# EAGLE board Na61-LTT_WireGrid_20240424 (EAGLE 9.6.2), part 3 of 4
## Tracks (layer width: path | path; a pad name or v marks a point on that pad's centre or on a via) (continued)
S$3176 (continued)
  Bottom 0.152: 35.8,85 36.2,85
S$3177
  Bottom 0.152: 36.2,85 37.2,86
S$3178
  Bottom 0.152: 33.8,85 34.6,85
S$3179
  Bottom 0.152: 34.6,85 35.6,86
S$3180
  Bottom 0.152: 40.8,89 41.2,89.4
S$3181
  Bottom 0.152: 41.2,89.4 41.2,90
S$3182
  Bottom 0.152: 38.8,89 39.6,89.8
S$3183
  Bottom 0.152: 39.6,89.8 39.6,90
S$3184
  Bottom 0.152: 36.8,89 37,89
S$3185
  Bottom 0.152: 37,89 38,90
S$3186
  Bottom 0.152: 34.8,89 35.4,89
S$3187
  Bottom 0.152: 35.4,89 36.4,90
S$3188
  Bottom 0.152: 32.8,87 33.8,86
S$3189
  Bottom 0.152: 33.8,86 34.8,86
S$3190
  Bottom 0.152: 34.6,91 34,91
S$3191
  Bottom 0.152: 34,91 33,90
S$3192
  Bottom 0.152: 33,90 32.4,90
S$3193
  Bottom 0.152: 32.6,91 31.6,90
S$3194
  Bottom 0.152: 31.6,90 30.8,90
S$3195
  Bottom 0.152: 30.6,91 29.6,90
S$3196
  Bottom 0.152: 29.6,90 29.2,90
S$3197
  Bottom 0.152: 28.6,91 27.6,90
S$3198
  Bottom 0.152: 26.6,91 26,90.4
S$3199
  Bottom 0.152: 26,90.4 26,90
S$3200
  Bottom 0.152: 35.6,95 34.6,94
S$3201
  Bottom 0.152: 34.6,94 33.2,94
S$3202
  Bottom 0.152: 33.6,95 33.2,95
S$3203
  Bottom 0.152: 33.2,95 32.2,94
S$3204
  Bottom 0.152: 32.2,94 31.6,94
S$3205
  Bottom 0.152: 31.6,95 31,95
S$3206
  Bottom 0.152: 31,95 30,94
S$3207
  Bottom 0.152: 29.6,95 29.4,95
S$3208
  Bottom 0.152: 29.4,95 28.4,94
S$3209
  Bottom 0.152: 27.6,95 26.8,94.2
S$3210
  Bottom 0.152: 26.8,94.2 26.8,94
S$3211
  Bottom 0.152: 34,90 35.2,90
S$3212
  Bottom 0.152: 35.2,90 36.2,91
S$3213
  Bottom 0.152: 36.2,91 36.6,91
S$3214  (2 unrouted)
  Top 0.813: 65,94.5 65,85.5
  Top 1.8: 66,91.5 64,91.5 | 66,94.5 65,94.5 64,94.5 | 66,88.5 64,88.5 | 66,85.5 65,85.5 64,85.5
S$3215
  Top 1.778: -104.08,86.83 -104.08,88.35
S$3216
  Top 1.778: -104.08,91.65 -104.08,93.17
S$3217
  Top 1.778: -99,86.83 -99,88.35
S$3218
  Top 1.778: -99,91.65 -99,93.17
S$3219
  Top 1.778: -93.92,86.83 -93.92,88.35
S$3220
  Top 1.778: -93.92,91.65 -93.92,93.17
S$3221
  Top 1.778: 93.92,86.83 93.92,88.35
S$3222
  Top 1.778: 93.92,91.65 93.92,93.17
S$3223
  Top 1.778: 99,86.83 99,88.35
S$3224
  Top 1.778: 99,91.65 99,93.17
S$3225
  Top 1.778: 104.08,86.83 104.08,88.35
S$3226
  Top 1.778: 104.08,91.65 104.08,93.17
S$3235
  Bottom 0.8: 9.4,102.9 9.4,101.1
S$3236
  Bottom 0.8: 11.4,102.9 11.4,101.1
S$3237
  Bottom 0.8: 8.4,105.1 8.4,106.9
S$3238
  Bottom 0.8: 10.4,105.1 10.4,106.9
S$3239
  Bottom 0.8: 5.4,102.9 5.4,101.1
S$3240
  Bottom 0.8: 7.4,102.9 7.4,101.1
S$3241
  Bottom 0.8: 6.4,105.1 6.4,106.9
S$3242
  Bottom 0.8: 4.4,105.1 4.4,106.9
S$3243
  Bottom 0.8: 3.4,102.9 3.4,101.1
S$3244
  Bottom 0.8: 1.4,102.9 1.4,101.1
S$3245
  Bottom 0.8: 2.4,105.1 2.4,106.9
S$3246
  Bottom 0.8: 0.4,105.1 0.4,106.9
S$3247
  Bottom 0.8: -0.6,102.9 -0.6,101.1
S$3248
  Bottom 0.8: -2.6,102.9 -2.6,101.1
S$3249
  Bottom 0.8: -1.6,105.1 -1.6,106.9
S$3250
  Bottom 0.8: 17.4,102.9 17.4,101.1
S$3251
  Bottom 0.8: 19.4,102.9 19.4,101.1
S$3252
  Bottom 0.8: 16.4,105.1 16.4,106.9
S$3253
  Bottom 0.8: 18.4,105.1 18.4,106.9
S$3254
  Bottom 0.8: 13.4,102.9 13.4,101.1
S$3255
  Bottom 0.8: 15.4,102.9 15.4,101.1
S$3256
  Bottom 0.8: 12.4,105.1 12.4,106.9
S$3257
  Bottom 0.8: 14.4,105.1 14.4,106.9
S$3258
  Bottom 0.8: -7.4,110.9 -7.4,109.1
S$3259
  Bottom 0.8: -5.4,110.9 -5.4,109.1
S$3260
  Bottom 0.8: -8.4,113.1 -8.4,114.9
S$3261
  Bottom 0.8: -6.4,113.1 -6.4,114.9
S$3262
  Bottom 0.8: -11.4,110.9 -11.4,109.1
S$3263
  Bottom 0.8: -9.4,110.9 -9.4,109.1
S$3264
  Bottom 0.8: -10.4,113.1 -10.4,114.9
S$3265
  Bottom 0.8: -12.4,113.1 -12.4,114.9
S$3266
  Bottom 0.8: -13.4,110.9 -13.4,109.1
S$3267
  Bottom 0.8: -15.4,110.9 -15.4,109.1
S$3268
  Bottom 0.8: -14.4,113.1 -14.4,114.9
S$3269
  Bottom 0.8: -16.4,113.1 -16.4,114.9
S$3270
  Bottom 0.8: -17.4,110.9 -17.4,109.1
S$3271
  Bottom 0.8: -19.4,110.9 -19.4,109.1
S$3272
  Bottom 0.8: -18.4,113.1 -18.4,114.9
S$3273
  Bottom 0.8: 0.6,110.9 0.6,109.1
S$3274
  Bottom 0.8: 2.6,110.9 2.6,109.1
S$3275
  Bottom 0.8: -0.4,113.1 -0.4,114.9
S$3276
  Bottom 0.8: 1.6,113.1 1.6,114.9
S$3277
  Bottom 0.8: -3.4,110.9 -3.4,109.1
S$3278
  Bottom 0.8: -1.4,110.9 -1.4,109.1
S$3279
  Bottom 0.8: -4.4,113.1 -4.4,114.9
S$3280
  Bottom 0.8: -2.4,113.1 -2.4,114.9
S$3281
  Bottom 0.8: -24.6,102.9 -24.6,101.1
S$3282
  Bottom 0.8: -22.6,102.9 -22.6,101.1
S$3283
  Bottom 0.8: -25.6,105.1 -25.6,106.9
S$3284
  Bottom 0.8: -23.6,105.1 -23.6,106.9
S$3285
  Bottom 0.8: -28.6,102.9 -28.6,101.1
S$3286
  Bottom 0.8: -26.6,102.9 -26.6,101.1
S$3287
  Bottom 0.8: -27.6,105.1 -27.6,106.9
S$3288
  Bottom 0.8: -29.6,105.1 -29.6,106.9
S$3289
  Bottom 0.8: -30.6,102.9 -30.6,101.1
S$3290
  Bottom 0.8: -32.6,102.9 -32.6,101.1
S$3291
  Bottom 0.8: -31.6,105.1 -31.6,106.9
S$3292
  Bottom 0.8: -33.6,105.1 -33.6,106.9
S$3293
  Bottom 0.8: -34.6,102.9 -34.6,101.1
S$3294
  Bottom 0.8: -36.6,102.9 -36.6,101.1
S$3295
  Bottom 0.8: -35.6,105.1 -35.6,106.9
S$3296
  Bottom 0.8: -16.6,102.9 -16.6,101.1
S$3297
  Bottom 0.8: -14.6,102.9 -14.6,101.1
S$3298
  Bottom 0.8: -17.6,105.1 -17.6,106.9
S$3299
  Bottom 0.8: -15.6,105.1 -15.6,106.9
S$3300
  Bottom 0.8: -20.6,102.9 -20.6,101.1
S$3301
  Bottom 0.8: -18.6,102.9 -18.6,101.1
S$3302
  Bottom 0.8: -21.6,105.1 -21.6,106.9
S$3303
  Bottom 0.8: -19.6,105.1 -19.6,106.9
S$3304
  Bottom 0.8: 26.6,110.9 26.6,109.1
S$3305
  Bottom 0.8: 28.6,110.9 28.6,109.1
S$3306
  Bottom 0.8: 25.6,113.1 25.6,114.9
S$3307
  Bottom 0.8: 27.6,113.1 27.6,114.9
S$3308
  Bottom 0.8: 22.6,110.9 22.6,109.1
S$3309
  Bottom 0.8: 24.6,110.9 24.6,109.1
S$3310
  Bottom 0.8: 23.6,113.1 23.6,114.9
S$3311
  Bottom 0.8: 21.6,113.1 21.6,114.9
S$3312
  Bottom 0.8: 20.6,110.9 20.6,109.1
S$3313
  Bottom 0.8: 18.6,110.9 18.6,109.1
S$3314
  Bottom 0.8: 19.6,113.1 19.6,114.9
S$3315
  Bottom 0.8: 17.6,113.1 17.6,114.9
S$3316
  Bottom 0.8: 16.6,110.9 16.6,109.1
S$3317
  Bottom 0.8: 14.6,110.9 14.6,109.1
S$3318
  Bottom 0.8: 15.6,113.1 15.6,114.9
S$3319
  Bottom 0.8: 34.6,110.9 34.6,109.1
S$3320
  Bottom 0.8: 36.6,110.9 36.6,109.1
S$3321
  Bottom 0.8: 33.6,113.1 33.6,114.9
S$3322
  Bottom 0.8: 35.6,113.1 35.6,114.9
S$3323
  Bottom 0.8: 30.6,110.9 30.6,109.1
S$3324
  Bottom 0.8: 32.6,110.9 32.6,109.1
S$3325
  Bottom 0.8: 29.6,113.1 29.6,114.9
S$3326
  Bottom 0.8: 31.6,113.1 31.6,114.9
S$3327
  Bottom 0.8: -41.8,110.9 -41.8,109.1
S$3328
  Bottom 0.8: -39.8,110.9 -39.8,109.1
S$3329
  Bottom 0.8: -42.8,113.1 -42.8,114.9
S$3330
  Bottom 0.8: -40.8,113.1 -40.8,114.9
S$3331
  Bottom 0.8: -45.8,110.9 -45.8,109.1
S$3332
  Bottom 0.8: -43.8,110.9 -43.8,109.1
S$3333
  Bottom 0.8: -44.8,113.1 -44.8,114.9
S$3334
  Bottom 0.8: -46.8,113.1 -46.8,114.9
S$3335
  Bottom 0.8: -47.8,110.9 -47.8,109.1
S$3336
  Bottom 0.8: -49.8,110.9 -49.8,109.1
S$3337
  Bottom 0.8: -48.8,113.1 -48.8,114.9
S$3338
  Bottom 0.8: -50.8,113.1 -50.8,114.9
S$3339
  Bottom 0.8: -51.8,110.9 -51.8,109.1
S$3340
  Bottom 0.8: -53.8,110.9 -53.8,109.1
S$3341
  Bottom 0.8: -52.8,113.1 -52.8,114.9
S$3342
  Bottom 0.8: -33.8,110.9 -33.8,109.1
S$3343
  Bottom 0.8: -31.8,110.9 -31.8,109.1
S$3344
  Bottom 0.8: -34.8,113.1 -34.8,114.9
S$3345
  Bottom 0.8: -32.8,113.1 -32.8,114.9
S$3346
  Bottom 0.8: -37.8,110.9 -37.8,109.1
S$3347
  Bottom 0.8: -35.8,110.9 -35.8,109.1
S$3348
  Bottom 0.8: -38.8,113.1 -38.8,114.9
S$3349
  Bottom 0.8: -36.8,113.1 -36.8,114.9
S$3350
  Bottom 0.8: 43.8,102.9 43.8,101.1
S$3351
  Bottom 0.8: 45.8,102.9 45.8,101.1
S$3352
  Bottom 0.8: 42.8,105.1 42.8,106.9
S$3353
  Bottom 0.8: 44.8,105.1 44.8,106.9
S$3354
  Bottom 0.8: 39.8,102.9 39.8,101.1
S$3355
  Bottom 0.8: 41.8,102.9 41.8,101.1
S$3356
  Bottom 0.8: 40.8,105.1 40.8,106.9
S$3357
  Bottom 0.8: 38.8,105.1 38.8,106.9
S$3358
  Bottom 0.8: 37.8,102.9 37.8,101.1
S$3359
  Bottom 0.8: 35.8,102.9 35.8,101.1
S$3360
  Bottom 0.8: 36.8,105.1 36.8,106.9
S$3361
  Bottom 0.8: 34.8,105.1 34.8,106.9
S$3362
  Bottom 0.8: 33.8,102.9 33.8,101.1
S$3363
  Bottom 0.8: 31.8,102.9 31.8,101.1
S$3364
  Bottom 0.8: 32.8,105.1 32.8,106.9
S$3365
  Bottom 0.8: 51.8,102.9 51.8,101.1
S$3366
  Bottom 0.8: 53.8,102.9 53.8,101.1
S$3367
  Bottom 0.8: 50.8,105.1 50.8,106.9
S$3368
  Bottom 0.8: 52.8,105.1 52.8,106.9
S$3369
  Bottom 0.8: 47.8,102.9 47.8,101.1
S$3370
  Bottom 0.8: 49.8,102.9 49.8,101.1
S$3371
  Bottom 0.8: 46.8,105.1 46.8,106.9
S$3372
  Bottom 0.8: 48.8,105.1 48.8,106.9
S$3501
  Bottom 0.152: -52.8,113 -51.8,112
S$3502
  Bottom 0.152: -51.8,112 -50.8,112
S$3503
  Bottom 0.152: -50.8,113 -50.2,113
S$3504
  Bottom 0.152: -50.2,113 -49.2,112
S$3505
  Bottom 0.152: -48.8,113 -48.6,113
S$3506
  Bottom 0.152: -48.6,113 -47.6,112
S$3507
  Bottom 0.152: -46.8,113 -46,112.2
S$3508
  Bottom 0.152: -46,112.2 -46,112
S$3509
  Bottom 0.152: -44.8,113 -44.4,112.6
S$3510
  Bottom 0.152: -44.4,112.6 -44.4,112
S$3511
  Bottom 0.152: -42.8,113 -42.8,112
S$3512
  Bottom 0.152: -40.8,113 -41.2,112.6
S$3513
  Bottom 0.152: -41.2,112.6 -41.2,112
S$3514
  Bottom 0.152: -38.8,113 -39.6,112.2
S$3515
  Bottom 0.152: -39.6,112.2 -39.6,112
S$3516
  Bottom 0.152: -36.8,113 -37,113
S$3517
  Bottom 0.152: -37,113 -38,112
S$3518
  Bottom 0.152: -34.8,113 -35.4,113
S$3519
  Bottom 0.152: -35.4,113 -36.4,112
S$3520
  Bottom 0.152: -32.8,113 -33.8,112
S$3521
  Bottom 0.152: -33.8,112 -34.8,112
S$3522
  Bottom 0.152: -51.8,109 -50.8,108
S$3523
  Bottom 0.152: -50.8,108 -50,108
S$3524
  Bottom 0.152: -49.8,109 -48.8,108
S$3525
  Bottom 0.152: -48.8,108 -48.4,108
S$3526
  Bottom 0.152: -47.8,109 -46.8,108
S$3527
  Bottom 0.152: -45.8,109 -45.2,108.4
S$3528
  Bottom 0.152: -45.2,108.4 -45.2,108
S$3529
  Bottom 0.152: -43.8,109 -43.6,108.8
S$3530
  Bottom 0.152: -43.6,108.8 -43.6,108
S$3531
  Bottom 0.152: -41.8,109 -42,108.8
S$3532
  Bottom 0.152: -42,108.8 -42,108
S$3533
  Bottom 0.152: -39.8,109 -40.4,108.4
S$3534
  Bottom 0.152: -40.4,108.4 -40.4,108
S$3535
  Bottom 0.152: -37.8,109 -38.8,108
S$3536
  Bottom 0.152: -35.8,109 -36.8,108
S$3537
  Bottom 0.152: -36.8,108 -37.2,108
S$3538
  Bottom 0.152: -33.8,109 -34.8,108
S$3539
  Bottom 0.152: -34.8,108 -35.6,108
S$3540
  Bottom 0.152: -36.6,103 -35.6,104
S$3541
  Bottom 0.152: -35.6,104 -34,104
S$3542
  Bottom 0.152: -34.6,103 -33.8,103
S$3543
  Bottom 0.152: -33.8,103 -32.8,104
S$3544
  Bottom 0.152: -32.8,104 -32.4,104
S$3545
  Bottom 0.152: -32.6,103 -31.8,103
S$3546
  Bottom 0.152: -31.8,103 -30.8,104
S$3547
  Bottom 0.152: -30.6,103 -30.2,103
S$3548
  Bottom 0.152: -30.2,103 -29.2,104
S$3549
  Bottom 0.152: -28.6,103 -27.6,104
S$3550
  Bottom 0.152: -26.6,103 -26,103.6
S$3551
  Bottom 0.152: -26,103.6 -26,104
S$3552
  Bottom 0.152: -35.6,107 -35,107
S$3553
  Bottom 0.152: -35,107 -34,108
S$3554
  Bottom 0.152: -34,108 -33.2,108
S$3555
  Bottom 0.152: -33.6,107 -33,107
S$3556
  Bottom 0.152: -33,107 -32,108
S$3557
  Bottom 0.152: -32,108 -31.6,108
S$3558
  Bottom 0.152: -31.6,107 -31,107
S$3559
  Bottom 0.152: -31,107 -30,108
S$3560
  Bottom 0.152: -29.6,107 -29.4,107
S$3561
  Bottom 0.152: -29.4,107 -28.4,108
S$3562
  Bottom 0.152: -27.6,107 -26.8,107.8
S$3563
  Bottom 0.152: -26.8,107.8 -26.8,108
S$3564
  Bottom 0.152: 1.6,113 0.6,112
S$3565
  Bottom 0.152: 0.6,112 -0.4,112
S$3566
  Bottom 0.152: -0.4,113 -1,113
S$3567
  Bottom 0.152: -1,113 -2,112
S$3568
  Bottom 0.152: -2.4,113 -2.6,113
S$3569
  Bottom 0.152: -2.6,113 -3.6,112
S$3570
  Bottom 0.152: -4.4,113 -5.2,112.2
S$3571
  Bottom 0.152: -5.2,112.2 -5.2,112
S$3572
  Bottom 0.152: -6.4,113 -6.8,112.6
S$3573
  Bottom 0.152: -6.8,112.6 -6.8,112
S$3574
  Bottom 0.152: -8.4,113 -8.4,112
S$3575
  Bottom 0.152: -10.4,113 -10,112.6
S$3576
  Bottom 0.152: -10,112.6 -10,112
S$3577
  Bottom 0.152: -12.4,113 -11.6,112.2
S$3578
  Bottom 0.152: -11.6,112.2 -11.6,112
S$3579
  Bottom 0.152: -14.4,113 -14.2,113
S$3580
  Bottom 0.152: -14.2,113 -13.2,112
S$3581
  Bottom 0.152: -16.4,113 -15.8,113
S$3582
  Bottom 0.152: -15.8,113 -14.8,112
S$3583
  Bottom 0.152: -18.4,113 -17.4,112
S$3584
  Bottom 0.152: -17.4,112 -16.4,112
S$3585
  Bottom 0.152: 0.6,109 -0.4,108
S$3586
  Bottom 0.152: -0.4,108 -1.2,108
S$3587
  Bottom 0.152: -1.4,109 -2.4,108
S$3588
  Bottom 0.152: -2.4,108 -2.8,108
S$3589
  Bottom 0.152: -3.4,109 -4.4,108
S$3590
  Bottom 0.152: -5.4,109 -6,108.4
S$3591
  Bottom 0.152: -6,108.4 -6,108
S$3592
  Bottom 0.152: -7.4,109 -7.6,108.8
S$3593
  Bottom 0.152: -7.6,108.8 -7.6,108
S$3594
  Bottom 0.152: -9.4,109 -9.2,108.8
S$3595
  Bottom 0.152: -9.2,108.8 -9.2,108
S$3596
  Bottom 0.152: -11.4,109 -10.8,108.4
S$3597
  Bottom 0.152: -10.8,108.4 -10.8,108
S$3598
  Bottom 0.152: -13.4,109 -12.4,108
S$3599
  Bottom 0.152: -15.4,109 -14.4,108
S$3600
  Bottom 0.152: -14.4,108 -14,108
S$3601
  Bottom 0.152: -17.4,109 -16.4,108
S$3602
  Bottom 0.152: -16.4,108 -15.6,108
S$3603
  Bottom 0.152: -14.6,103 -15.6,104
S$3604
  Bottom 0.152: -15.6,104 -17.2,104
S$3605
  Bottom 0.152: -16.6,103 -17.4,103
S$3606
  Bottom 0.152: -17.4,103 -18.4,104
S$3607
  Bottom 0.152: -18.4,104 -18.8,104
S$3608
  Bottom 0.152: -18.6,103 -19.4,103
S$3609
  Bottom 0.152: -19.4,103 -20.4,104
S$3610
  Bottom 0.152: -20.6,103 -21,103
S$3611
  Bottom 0.152: -21,103 -22,104
S$3612
  Bottom 0.152: -22.6,103 -23.6,104
S$3613
  Bottom 0.152: -24.6,103 -25.2,103.6
S$3614
  Bottom 0.152: -25.2,103.6 -25.2,104
S$3615
  Bottom 0.152: -15.6,107 -16.2,107
S$3616
  Bottom 0.152: -16.2,107 -17.2,108
S$3617
  Bottom 0.152: -17.2,108 -18,108
S$3618
  Bottom 0.152: -17.6,107 -18.2,107
S$3619
  Bottom 0.152: -18.2,107 -19.2,108
S$3620
  Bottom 0.152: -19.2,108 -19.6,108
S$3621
  Bottom 0.152: -19.6,107 -20.2,107
S$3622
  Bottom 0.152: -20.2,107 -21.2,108
S$3623
  Bottom 0.152: -21.6,107 -21.8,107
S$3624
  Bottom 0.152: -21.8,107 -22.8,108
S$3625
  Bottom 0.152: -23.6,107 -24.4,107.8
S$3626
  Bottom 0.152: -24.4,107.8 -24.4,108
S$3627
  Bottom 0.152: 0.4,107 1,107
S$3628
  Bottom 0.152: 1,107 2,108
S$3629
  Bottom 0.152: 2.4,107 2.6,107
S$3630
  Bottom 0.152: 2.6,107 3.6,108
S$3631
  Bottom 0.152: 4.4,107 5.2,107.8
S$3632
  Bottom 0.152: 5.2,107.8 5.2,108
S$3633
  Bottom 0.152: 6.4,107 6.8,107.4
S$3634
  Bottom 0.152: 6.8,107.4 6.8,108
S$3635
  Bottom 0.152: 8.4,107 8.4,108
S$3636
  Bottom 0.152: -1.6,107 -0.6,107
S$3637
  Bottom 0.152: -0.6,107 0.4,108
S$3638
  Bottom 0.152: -0.6,103 0.4,104
S$3639
  Bottom 0.152: 0.4,104 1.2,104
S$3640
  Bottom 0.152: 1.4,103 1.8,103
S$3641
  Bottom 0.152: 1.8,103 2.8,104
S$3642
  Bottom 0.152: 3.4,103 4.4,104
S$3643
  Bottom 0.152: 5.4,103 6,103.6
S$3644
  Bottom 0.152: 6,103.6 6,104
S$3645
  Bottom 0.152: 7.4,103 7.6,103.2
S$3646
  Bottom 0.152: 7.6,103.2 7.6,104
S$3647
  Bottom 0.152: 9.4,103 9.2,103.2
S$3648
  Bottom 0.152: 9.2,103.2 9.2,104
S$3649
  Bottom 0.152: 11.4,103 10.8,103.6
S$3650
  Bottom 0.152: 10.8,103.6 10.8,104
S$3651
  Bottom 0.152: 13.4,103 12.4,104
S$3652
  Bottom 0.152: 15.4,103 15,103
S$3653
  Bottom 0.152: 15,103 14,104
S$3654
  Bottom 0.152: 17.4,103 16.6,103
S$3655
  Bottom 0.152: 16.6,103 15.6,104
S$3656
  Bottom 0.152: 10.4,107 10,107.4
S$3657
  Bottom 0.152: 10,107.4 10,108
S$3658
  Bottom 0.152: 12.4,107 11.6,107.8
S$3659
  Bottom 0.152: 11.6,107.8 11.6,108
S$3660
  Bottom 0.152: 14.4,107 14.2,107
S$3661
  Bottom 0.152: 14.2,107 13.2,108
S$3662
  Bottom 0.152: 16.4,107 15.8,107
S$3663
  Bottom 0.152: 15.8,107 14.8,108
S$3664
  Bottom 0.152: 18.4,105 17.4,104
S$3665
  Bottom 0.152: 17.4,104 16.4,104
S$3666
  Bottom 0.152: 16.6,109 17.2,109
S$3667
  Bottom 0.152: 17.2,109 18.2,108
S$3668
  Bottom 0.152: 18.2,108 18.8,108
S$3669
  Bottom 0.152: 18.6,109 19.6,108
S$3670
  Bottom 0.152: 19.6,108 20.4,108
S$3671
  Bottom 0.152: 20.6,109 21.6,108
S$3672
  Bottom 0.152: 21.6,108 22,108
S$3673
  Bottom 0.152: 22.6,109 23.6,108
S$3674
  Bottom 0.152: 24.6,109 25.2,108.4
S$3675
  Bottom 0.152: 25.2,108.4 25.2,108
S$3676
  Bottom 0.152: 15.6,113 16.6,112
S$3677
  Bottom 0.152: 16.6,112 18,112
S$3678
  Bottom 0.152: 17.6,113 18,113
S$3679
  Bottom 0.152: 18,113 19,112
S$3680
  Bottom 0.152: 19,112 19.6,112
S$3681
  Bottom 0.152: 19.6,113 20.2,113
S$3682
  Bottom 0.152: 20.2,113 21.2,112
S$3683
  Bottom 0.152: 21.6,113 21.8,113
S$3684
  Bottom 0.152: 21.8,113 22.8,112
S$3685
  Bottom 0.152: 23.6,113 24.4,112.2
S$3686
  Bottom 0.152: 24.4,112.2 24.4,112
S$3687
  Bottom 0.152: 17.2,108 16,108
S$3688
  Bottom 0.152: 16,108 15,109
S$3689
  Bottom 0.152: 15,109 14.6,109
S$3690
  Bottom 0.152: 50.8,107 50.2,107
S$3691
  Bottom 0.152: 50.2,107 49.2,108
S$3692
  Bottom 0.152: 48.8,107 48.6,107
S$3693
  Bottom 0.152: 48.6,107 47.6,108
S$3694
  Bottom 0.152: 46.8,107 46,107.8
S$3695
  Bottom 0.152: 46,107.8 46,108
S$3696
  Bottom 0.152: 44.8,107 44.4,107.4
S$3697
  Bottom 0.152: 44.4,107.4 44.4,108
S$3698
  Bottom 0.152: 42.8,107 42.8,108
S$3699
  Bottom 0.152: 52.8,107 51.8,107
S$3700
  Bottom 0.152: 51.8,107 50.8,108
S$3701
  Bottom 0.152: 51.8,103 50.8,104
S$3702
  Bottom 0.152: 50.8,104 50,104
S$3703
  Bottom 0.152: 49.8,103 49.4,103
S$3704
  Bottom 0.152: 49.4,103 48.4,104
S$3705
  Bottom 0.152: 47.8,103 46.8,104
S$3706
  Bottom 0.152: 45.8,103 45.2,103.6
S$3707
  Bottom 0.152: 45.2,103.6 45.2,104
S$3708
  Bottom 0.152: 43.8,103 43.6,103.2
S$3709
  Bottom 0.152: 43.6,103.2 43.6,104
S$3710
  Bottom 0.152: 41.8,103 42,103.2
S$3711
  Bottom 0.152: 42,103.2 42,104
S$3712
  Bottom 0.152: 39.8,103 40.4,103.6
S$3713
  Bottom 0.152: 40.4,103.6 40.4,104
S$3714
  Bottom 0.152: 37.8,103 38.8,104
S$3715
  Bottom 0.152: 35.8,103 36.2,103
S$3716
  Bottom 0.152: 36.2,103 37.2,104
S$3717
  Bottom 0.152: 33.8,103 34.6,103
S$3718
  Bottom 0.152: 34.6,103 35.6,104
S$3719
  Bottom 0.152: 40.8,107 41.2,107.4
S$3720
  Bottom 0.152: 41.2,107.4 41.2,108
S$3721
  Bottom 0.152: 38.8,107 39.6,107.8
S$3722
  Bottom 0.152: 39.6,107.8 39.6,108
S$3723
  Bottom 0.152: 36.8,107 37,107
S$3724
  Bottom 0.152: 37,107 38,108
S$3725
  Bottom 0.152: 34.8,107 35.4,107
S$3726
  Bottom 0.152: 35.4,107 36.4,108
S$3727
  Bottom 0.152: 32.8,105 33.8,104
S$3728
  Bottom 0.152: 33.8,104 34.8,104
S$3729
  Bottom 0.152: 34.6,109 34,109
S$3730
  Bottom 0.152: 34,109 33,108
S$3731
  Bottom 0.152: 33,108 32.4,108
S$3732
  Bottom 0.152: 32.6,109 31.6,108
S$3733
  Bottom 0.152: 31.6,108 30.8,108
S$3734
  Bottom 0.152: 30.6,109 29.6,108
S$3735
  Bottom 0.152: 29.6,108 29.2,108
S$3736
  Bottom 0.152: 28.6,109 27.6,108
S$3737
  Bottom 0.152: 26.6,109 26,108.4
S$3738
  Bottom 0.152: 26,108.4 26,108
S$3739
  Bottom 0.152: 35.6,113 34.6,112
S$3740
  Bottom 0.152: 34.6,112 33.2,112
S$3741
  Bottom 0.152: 33.6,113 33.2,113
S$3742
  Bottom 0.152: 33.2,113 32.2,112
S$3743
  Bottom 0.152: 32.2,112 31.6,112
S$3744
  Bottom 0.152: 31.6,113 31,113
S$3745
  Bottom 0.152: 31,113 30,112
S$3746
  Bottom 0.152: 29.6,113 29.4,113
S$3747
  Bottom 0.152: 29.4,113 28.4,112
S$3748
  Bottom 0.152: 27.6,113 26.8,112.2
S$3749
  Bottom 0.152: 26.8,112.2 26.8,112
S$3750
  Bottom 0.152: 34,108 35.2,108
S$3751
  Bottom 0.152: 35.2,108 36.2,109
S$3752
  Bottom 0.152: 36.2,109 36.6,109
S$3753  (2 unrouted)
  Top 0.813: 65,112.5 65,103.5
  Top 1.8: 66,109.5 64,109.5 | 66,112.5 65,112.5 64,112.5 | 66,106.5 64,106.5 | 66,103.5 65,103.5 64,103.5
S$3754
  Top 1.778: -104.08,104.83 -104.08,106.35
S$3755
  Top 1.778: -104.08,109.65 -104.08,111.17
S$3756
  Top 1.778: -99,104.83 -99,106.35
S$3757
  Top 1.778: -99,109.65 -99,111.17
S$3758
  Top 1.778: -93.92,104.83 -93.92,106.35
S$3759
  Top 1.778: -93.92,109.65 -93.92,111.17
S$3760
  Top 1.778: 93.92,104.83 93.92,106.35
S$3761
  Top 1.778: 93.92,109.65 93.92,111.17
S$3762
  Top 1.778: 99,104.83 99,106.35
S$3763
  Top 1.778: 99,109.65 99,111.17
S$3764
  Top 1.778: 104.08,104.83 104.08,106.35
S$3765
  Top 1.778: 104.08,109.65 104.08,111.17
S$3774
  Bottom 0.8: 9.4,120.9 9.4,119.1
S$3775
  Bottom 0.8: 11.4,120.9 11.4,119.1
S$3776
  Bottom 0.8: 8.4,123.1 8.4,124.9
S$3777
  Bottom 0.8: 10.4,123.1 10.4,124.9
S$3778
  Bottom 0.8: 5.4,120.9 5.4,119.1
S$3779
  Bottom 0.8: 7.4,120.9 7.4,119.1
S$3780
  Bottom 0.8: 6.4,123.1 6.4,124.9
S$3781
  Bottom 0.8: 4.4,123.1 4.4,124.9
S$3782
  Bottom 0.8: 3.4,120.9 3.4,119.1
S$3783
  Bottom 0.8: 1.4,120.9 1.4,119.1
S$3784
  Bottom 0.8: 2.4,123.1 2.4,124.9
S$3785
  Bottom 0.8: 0.4,123.1 0.4,124.9
S$3786
  Bottom 0.8: -0.6,120.9 -0.6,119.1
S$3787
  Bottom 0.8: -2.6,120.9 -2.6,119.1
S$3788
  Bottom 0.8: -1.6,123.1 -1.6,124.9
S$3789
  Bottom 0.8: 17.4,120.9 17.4,119.1
S$3790
  Bottom 0.8: 19.4,120.9 19.4,119.1
S$3791
  Bottom 0.8: 16.4,123.1 16.4,124.9
S$3792
  Bottom 0.8: 18.4,123.1 18.4,124.9
S$3793
  Bottom 0.8: 13.4,120.9 13.4,119.1
S$3794
  Bottom 0.8: 15.4,120.9 15.4,119.1
S$3795
  Bottom 0.8: 12.4,123.1 12.4,124.9
S$3796
  Bottom 0.8: 14.4,123.1 14.4,124.9
S$3797
  Bottom 0.8: -7.4,128.9 -7.4,127.1
S$3798
  Bottom 0.8: -5.4,128.9 -5.4,127.1
S$3799
  Bottom 0.8: -8.4,131.1 -8.4,132.9
S$3800
  Bottom 0.8: -6.4,131.1 -6.4,132.9
S$3801
  Bottom 0.8: -11.4,128.9 -11.4,127.1
S$3802
  Bottom 0.8: -9.4,128.9 -9.4,127.1
S$3803
  Bottom 0.8: -10.4,131.1 -10.4,132.9
S$3804
  Bottom 0.8: -12.4,131.1 -12.4,132.9
S$3805
  Bottom 0.8: -13.4,128.9 -13.4,127.1
S$3806
  Bottom 0.8: -15.4,128.9 -15.4,127.1
S$3807
  Bottom 0.8: -14.4,131.1 -14.4,132.9
S$3808
  Bottom 0.8: -16.4,131.1 -16.4,132.9
S$3809
  Bottom 0.8: -17.4,128.9 -17.4,127.1
S$3810
  Bottom 0.8: -19.4,128.9 -19.4,127.1
S$3811
  Bottom 0.8: -18.4,131.1 -18.4,132.9
S$3812
  Bottom 0.8: 0.6,128.9 0.6,127.1
S$3813
  Bottom 0.8: 2.6,128.9 2.6,127.1
S$3814
  Bottom 0.8: -0.4,131.1 -0.4,132.9
S$3815
  Bottom 0.8: 1.6,131.1 1.6,132.9
S$3816
  Bottom 0.8: -3.4,128.9 -3.4,127.1
S$3817
  Bottom 0.8: -1.4,128.9 -1.4,127.1
S$3818
  Bottom 0.8: -4.4,131.1 -4.4,132.9
S$3819
  Bottom 0.8: -2.4,131.1 -2.4,132.9
S$3820
  Bottom 0.8: -24.6,120.9 -24.6,119.1
S$3821
  Bottom 0.8: -22.6,120.9 -22.6,119.1
S$3822
  Bottom 0.8: -25.6,123.1 -25.6,124.9
S$3823
  Bottom 0.8: -23.6,123.1 -23.6,124.9
S$3824
  Bottom 0.8: -28.6,120.9 -28.6,119.1
S$3825
  Bottom 0.8: -26.6,120.9 -26.6,119.1
S$3826
  Bottom 0.8: -27.6,123.1 -27.6,124.9
S$3827
  Bottom 0.8: -29.6,123.1 -29.6,124.9
S$3828
  Bottom 0.8: -30.6,120.9 -30.6,119.1
S$3829
  Bottom 0.8: -32.6,120.9 -32.6,119.1
S$3830
  Bottom 0.8: -31.6,123.1 -31.6,124.9
S$3831
  Bottom 0.8: -33.6,123.1 -33.6,124.9
S$3832
  Bottom 0.8: -34.6,120.9 -34.6,119.1
S$3833
  Bottom 0.8: -36.6,120.9 -36.6,119.1
S$3834
  Bottom 0.8: -35.6,123.1 -35.6,124.9
S$3835
  Bottom 0.8: -16.6,120.9 -16.6,119.1
S$3836
  Bottom 0.8: -14.6,120.9 -14.6,119.1
S$3837
  Bottom 0.8: -17.6,123.1 -17.6,124.9
S$3838
  Bottom 0.8: -15.6,123.1 -15.6,124.9
S$3839
  Bottom 0.8: -20.6,120.9 -20.6,119.1
S$3840
  Bottom 0.8: -18.6,120.9 -18.6,119.1
S$3841
  Bottom 0.8: -21.6,123.1 -21.6,124.9
S$3842
  Bottom 0.8: -19.6,123.1 -19.6,124.9
S$3843
  Bottom 0.8: 26.6,128.9 26.6,127.1
S$3844
  Bottom 0.8: 28.6,128.9 28.6,127.1
S$3845
  Bottom 0.8: 25.6,131.1 25.6,132.9
S$3846
  Bottom 0.8: 27.6,131.1 27.6,132.9
S$3847
  Bottom 0.8: 22.6,128.9 22.6,127.1
S$3848
  Bottom 0.8: 24.6,128.9 24.6,127.1
S$3849
  Bottom 0.8: 23.6,131.1 23.6,132.9
S$3850
  Bottom 0.8: 21.6,131.1 21.6,132.9
S$3851
  Bottom 0.8: 20.6,128.9 20.6,127.1
S$3852
  Bottom 0.8: 18.6,128.9 18.6,127.1
S$3853
  Bottom 0.8: 19.6,131.1 19.6,132.9
S$3854
  Bottom 0.8: 17.6,131.1 17.6,132.9
S$3855
  Bottom 0.8: 16.6,128.9 16.6,127.1
S$3856
  Bottom 0.8: 14.6,128.9 14.6,127.1
S$3857
  Bottom 0.8: 15.6,131.1 15.6,132.9
S$3858
  Bottom 0.8: 34.6,128.9 34.6,127.1
S$3859
  Bottom 0.8: 36.6,128.9 36.6,127.1
S$3860
  Bottom 0.8: 33.6,131.1 33.6,132.9
S$3861
  Bottom 0.8: 35.6,131.1 35.6,132.9
S$3862
  Bottom 0.8: 30.6,128.9 30.6,127.1
S$3863
  Bottom 0.8: 32.6,128.9 32.6,127.1
S$3864
  Bottom 0.8: 29.6,131.1 29.6,132.9
S$3865
  Bottom 0.8: 31.6,131.1 31.6,132.9
S$3866
  Bottom 0.8: -41.8,128.9 -41.8,127.1
S$3867
  Bottom 0.8: -39.8,128.9 -39.8,127.1
S$3868
  Bottom 0.8: -42.8,131.1 -42.8,132.9
S$3869
  Bottom 0.8: -40.8,131.1 -40.8,132.9
S$3870
  Bottom 0.8: -45.8,128.9 -45.8,127.1
S$3871
  Bottom 0.8: -43.8,128.9 -43.8,127.1
S$3872
  Bottom 0.8: -44.8,131.1 -44.8,132.9
S$3873
  Bottom 0.8: -46.8,131.1 -46.8,132.9
S$3874
  Bottom 0.8: -47.8,128.9 -47.8,127.1
S$3875
  Bottom 0.8: -49.8,128.9 -49.8,127.1
S$3876
  Bottom 0.8: -48.8,131.1 -48.8,132.9
S$3877
  Bottom 0.8: -50.8,131.1 -50.8,132.9
S$3878
  Bottom 0.8: -51.8,128.9 -51.8,127.1
S$3879
  Bottom 0.8: -53.8,128.9 -53.8,127.1
S$3880
  Bottom 0.8: -52.8,131.1 -52.8,132.9
S$3881
  Bottom 0.8: -33.8,128.9 -33.8,127.1
S$3882
  Bottom 0.8: -31.8,128.9 -31.8,127.1
S$3883
  Bottom 0.8: -34.8,131.1 -34.8,132.9
S$3884
  Bottom 0.8: -32.8,131.1 -32.8,132.9
S$3885
  Bottom 0.8: -37.8,128.9 -37.8,127.1
S$3886
  Bottom 0.8: -35.8,128.9 -35.8,127.1
S$3887
  Bottom 0.8: -38.8,131.1 -38.8,132.9
S$3888
  Bottom 0.8: -36.8,131.1 -36.8,132.9
S$3889
  Bottom 0.8: 43.8,120.9 43.8,119.1
S$3890
  Bottom 0.8: 45.8,120.9 45.8,119.1
S$3891
  Bottom 0.8: 42.8,123.1 42.8,124.9
S$3892
  Bottom 0.8: 44.8,123.1 44.8,124.9
S$3893
  Bottom 0.8: 39.8,120.9 39.8,119.1
S$3894
  Bottom 0.8: 41.8,120.9 41.8,119.1
S$3895
  Bottom 0.8: 40.8,123.1 40.8,124.9
S$3896
  Bottom 0.8: 38.8,123.1 38.8,124.9
S$3897
  Bottom 0.8: 37.8,120.9 37.8,119.1
S$3898
  Bottom 0.8: 35.8,120.9 35.8,119.1
S$3899
  Bottom 0.8: 36.8,123.1 36.8,124.9
S$3900
  Bottom 0.8: 34.8,123.1 34.8,124.9
S$3901
  Bottom 0.8: 33.8,120.9 33.8,119.1
S$3902
  Bottom 0.8: 31.8,120.9 31.8,119.1
S$3903
  Bottom 0.8: 32.8,123.1 32.8,124.9
S$3904
  Bottom 0.8: 51.8,120.9 51.8,119.1
S$3905
  Bottom 0.8: 53.8,120.9 53.8,119.1
S$3906
  Bottom 0.8: 50.8,123.1 50.8,124.9
S$3907
  Bottom 0.8: 52.8,123.1 52.8,124.9
S$3908
  Bottom 0.8: 47.8,120.9 47.8,119.1
S$3909
  Bottom 0.8: 49.8,120.9 49.8,119.1
S$3910
  Bottom 0.8: 46.8,123.1 46.8,124.9
S$3911
  Bottom 0.8: 48.8,123.1 48.8,124.9
S$4040
  Bottom 0.152: -52.8,131 -51.8,130
S$4041
  Bottom 0.152: -51.8,130 -50.8,130
S$4042
  Bottom 0.152: -50.8,131 -50.2,131
S$4043
  Bottom 0.152: -50.2,131 -49.2,130
S$4044
  Bottom 0.152: -48.8,131 -48.6,131
S$4045
  Bottom 0.152: -48.6,131 -47.6,130
S$4046
  Bottom 0.152: -46.8,131 -46,130.2
S$4047
  Bottom 0.152: -46,130.2 -46,130
S$4048
  Bottom 0.152: -44.8,131 -44.4,130.6
S$4049
  Bottom 0.152: -44.4,130.6 -44.4,130
S$4050
  Bottom 0.152: -42.8,131 -42.8,130
S$4051
  Bottom 0.152: -40.8,131 -41.2,130.6
S$4052
  Bottom 0.152: -41.2,130.6 -41.2,130
S$4053
  Bottom 0.152: -38.8,131 -39.6,130.2
S$4054
  Bottom 0.152: -39.6,130.2 -39.6,130
S$4055
  Bottom 0.152: -36.8,131 -37,131
S$4056
  Bottom 0.152: -37,131 -38,130
S$4057
  Bottom 0.152: -34.8,131 -35.4,131
S$4058
  Bottom 0.152: -35.4,131 -36.4,130
S$4059
  Bottom 0.152: -32.8,131 -33.8,130
S$4060
  Bottom 0.152: -33.8,130 -34.8,130
S$4061
  Bottom 0.152: -51.8,127 -50.8,126
S$4062
  Bottom 0.152: -50.8,126 -50,126
S$4063
  Bottom 0.152: -49.8,127 -48.8,126
S$4064
  Bottom 0.152: -48.8,126 -48.4,126
S$4065
  Bottom 0.152: -47.8,127 -46.8,126
S$4066
  Bottom 0.152: -45.8,127 -45.2,126.4
S$4067
  Bottom 0.152: -45.2,126.4 -45.2,126
S$4068
  Bottom 0.152: -43.8,127 -43.6,126.8
S$4069
  Bottom 0.152: -43.6,126.8 -43.6,126
S$4070
  Bottom 0.152: -41.8,127 -42,126.8
S$4071
  Bottom 0.152: -42,126.8 -42,126
S$4072
  Bottom 0.152: -39.8,127 -40.4,126.4
S$4073
  Bottom 0.152: -40.4,126.4 -40.4,126
S$4074
  Bottom 0.152: -37.8,127 -38.8,126
S$4075
  Bottom 0.152: -35.8,127 -36.8,126
S$4076
  Bottom 0.152: -36.8,126 -37.2,126
S$4077
  Bottom 0.152: -33.8,127 -34.8,126
S$4078
  Bottom 0.152: -34.8,126 -35.6,126
S$4079
  Bottom 0.152: -36.6,121 -35.6,122
S$4080
  Bottom 0.152: -35.6,122 -34,122
S$4081
  Bottom 0.152: -34.6,121 -33.8,121
S$4082
  Bottom 0.152: -33.8,121 -32.8,122
S$4083
  Bottom 0.152: -32.8,122 -32.4,122
S$4084
  Bottom 0.152: -32.6,121 -31.8,121
S$4085
  Bottom 0.152: -31.8,121 -30.8,122
S$4086
  Bottom 0.152: -30.6,121 -30.2,121
S$4087
  Bottom 0.152: -30.2,121 -29.2,122
S$4088
  Bottom 0.152: -28.6,121 -27.6,122
S$4089
  Bottom 0.152: -26.6,121 -26,121.6
S$4090
  Bottom 0.152: -26,121.6 -26,122
S$4091
  Bottom 0.152: -35.6,125 -35,125
S$4092
  Bottom 0.152: -35,125 -34,126
S$4093
  Bottom 0.152: -34,126 -33.2,126
S$4094
  Bottom 0.152: -33.6,125 -33,125
S$4095
  Bottom 0.152: -33,125 -32,126
S$4096
  Bottom 0.152: -32,126 -31.6,126
S$4097
  Bottom 0.152: -31.6,125 -31,125
S$4098
  Bottom 0.152: -31,125 -30,126
S$4099
  Bottom 0.152: -29.6,125 -29.4,125
S$4100
  Bottom 0.152: -29.4,125 -28.4,126
S$4101
  Bottom 0.152: -27.6,125 -26.8,125.8
S$4102
  Bottom 0.152: -26.8,125.8 -26.8,126
S$4103
  Bottom 0.152: 1.6,131 0.6,130
S$4104
  Bottom 0.152: 0.6,130 -0.4,130
S$4105
  Bottom 0.152: -0.4,131 -1,131
S$4106
  Bottom 0.152: -1,131 -2,130
S$4107
  Bottom 0.152: -2.4,131 -2.6,131
S$4108
  Bottom 0.152: -2.6,131 -3.6,130
S$4109
  Bottom 0.152: -4.4,131 -5.2,130.2
S$4110
  Bottom 0.152: -5.2,130.2 -5.2,130
S$4111
  Bottom 0.152: -6.4,131 -6.8,130.6
S$4112
  Bottom 0.152: -6.8,130.6 -6.8,130
S$4113
  Bottom 0.152: -8.4,131 -8.4,130
S$4114
  Bottom 0.152: -10.4,131 -10,130.6
S$4115
  Bottom 0.152: -10,130.6 -10,130
S$4116
  Bottom 0.152: -12.4,131 -11.6,130.2
S$4117
  Bottom 0.152: -11.6,130.2 -11.6,130
S$4118
  Bottom 0.152: -14.4,131 -14.2,131
S$4119
  Bottom 0.152: -14.2,131 -13.2,130
S$4120
  Bottom 0.152: -16.4,131 -15.8,131
S$4121
  Bottom 0.152: -15.8,131 -14.8,130
S$4122
  Bottom 0.152: -18.4,131 -17.4,130
S$4123
  Bottom 0.152: -17.4,130 -16.4,130
S$4124
  Bottom 0.152: 0.6,127 -0.4,126
S$4125
  Bottom 0.152: -0.4,126 -1.2,126
S$4126
  Bottom 0.152: -1.4,127 -2.4,126
S$4127
  Bottom 0.152: -2.4,126 -2.8,126
S$4128
  Bottom 0.152: -3.4,127 -4.4,126
S$4129
  Bottom 0.152: -5.4,127 -6,126.4
S$4130
  Bottom 0.152: -6,126.4 -6,126
S$4131
  Bottom 0.152: -7.4,127 -7.6,126.8
S$4132
  Bottom 0.152: -7.6,126.8 -7.6,126
S$4133
  Bottom 0.152: -9.4,127 -9.2,126.8
S$4134
  Bottom 0.152: -9.2,126.8 -9.2,126
S$4135
  Bottom 0.152: -11.4,127 -10.8,126.4
S$4136
  Bottom 0.152: -10.8,126.4 -10.8,126
S$4137
  Bottom 0.152: -13.4,127 -12.4,126
S$4138
  Bottom 0.152: -15.4,127 -14.4,126
S$4139
  Bottom 0.152: -14.4,126 -14,126
S$4140
  Bottom 0.152: -17.4,127 -16.4,126
S$4141
  Bottom 0.152: -16.4,126 -15.6,126
S$4142
  Bottom 0.152: -14.6,121 -15.6,122
S$4143
  Bottom 0.152: -15.6,122 -17.2,122
S$4144
  Bottom 0.152: -16.6,121 -17.4,121
S$4145
  Bottom 0.152: -17.4,121 -18.4,122
S$4146
  Bottom 0.152: -18.4,122 -18.8,122
S$4147
  Bottom 0.152: -18.6,121 -19.4,121
S$4148
  Bottom 0.152: -19.4,121 -20.4,122
S$4149
  Bottom 0.152: -20.6,121 -21,121
S$4150
  Bottom 0.152: -21,121 -22,122
S$4151
  Bottom 0.152: -22.6,121 -23.6,122
S$4152
  Bottom 0.152: -24.6,121 -25.2,121.6
S$4153
  Bottom 0.152: -25.2,121.6 -25.2,122
S$4154
  Bottom 0.152: -15.6,125 -16.2,125
S$4155
  Bottom 0.152: -16.2,125 -17.2,126
S$4156
  Bottom 0.152: -17.2,126 -18,126
S$4157
  Bottom 0.152: -17.6,125 -18.2,125
S$4158
  Bottom 0.152: -18.2,125 -19.2,126
S$4159
  Bottom 0.152: -19.2,126 -19.6,126
S$4160
  Bottom 0.152: -19.6,125 -20.2,125
S$4161
  Bottom 0.152: -20.2,125 -21.2,126
S$4162
  Bottom 0.152: -21.6,125 -21.8,125
S$4163
  Bottom 0.152: -21.8,125 -22.8,126
S$4164
  Bottom 0.152: -23.6,125 -24.4,125.8
S$4165
  Bottom 0.152: -24.4,125.8 -24.4,126
S$4166
  Bottom 0.152: 0.4,125 1,125
S$4167
  Bottom 0.152: 1,125 2,126
S$4168
  Bottom 0.152: 2.4,125 2.6,125
S$4169
  Bottom 0.152: 2.6,125 3.6,126
S$4170
  Bottom 0.152: 4.4,125 5.2,125.8
S$4171
  Bottom 0.152: 5.2,125.8 5.2,126
S$4172
  Bottom 0.152: 6.4,125 6.8,125.4
S$4173
  Bottom 0.152: 6.8,125.4 6.8,126
S$4174
  Bottom 0.152: 8.4,125 8.4,126
S$4175
  Bottom 0.152: -1.6,125 -0.6,125
S$4176
  Bottom 0.152: -0.6,125 0.4,126
S$4177
  Bottom 0.152: -0.6,121 0.4,122
S$4178
  Bottom 0.152: 0.4,122 1.2,122
S$4179
  Bottom 0.152: 1.4,121 1.8,121
S$4180
  Bottom 0.152: 1.8,121 2.8,122
S$4181
  Bottom 0.152: 3.4,121 4.4,122
S$4182
  Bottom 0.152: 5.4,121 6,121.6
S$4183
  Bottom 0.152: 6,121.6 6,122
S$4184
  Bottom 0.152: 7.4,121 7.6,121.2
S$4185
  Bottom 0.152: 7.6,121.2 7.6,122
S$4186
  Bottom 0.152: 9.4,121 9.2,121.2
S$4187
  Bottom 0.152: 9.2,121.2 9.2,122
S$4188
  Bottom 0.152: 11.4,121 10.8,121.6
S$4189
  Bottom 0.152: 10.8,121.6 10.8,122
S$4190
  Bottom 0.152: 13.4,121 12.4,122
S$4191
  Bottom 0.152: 15.4,121 15,121
S$4192
  Bottom 0.152: 15,121 14,122
S$4193
  Bottom 0.152: 17.4,121 16.6,121
S$4194
  Bottom 0.152: 16.6,121 15.6,122
S$4195
  Bottom 0.152: 10.4,125 10,125.4
S$4196
  Bottom 0.152: 10,125.4 10,126
S$4197
  Bottom 0.152: 12.4,125 11.6,125.8
S$4198
  Bottom 0.152: 11.6,125.8 11.6,126
S$4199
  Bottom 0.152: 14.4,125 14.2,125
S$4200
  Bottom 0.152: 14.2,125 13.2,126
S$4201
  Bottom 0.152: 16.4,125 15.8,125
S$4202
  Bottom 0.152: 15.8,125 14.8,126
S$4203
  Bottom 0.152: 18.4,123 17.4,122
S$4204
  Bottom 0.152: 17.4,122 16.4,122
S$4205
  Bottom 0.152: 16.6,127 17.2,127
S$4206
  Bottom 0.152: 17.2,127 18.2,126
S$4207
  Bottom 0.152: 18.2,126 18.8,126
S$4208
  Bottom 0.152: 18.6,127 19.6,126
S$4209
  Bottom 0.152: 19.6,126 20.4,126
S$4210
  Bottom 0.152: 20.6,127 21.6,126
S$4211
  Bottom 0.152: 21.6,126 22,126
S$4212
  Bottom 0.152: 22.6,127 23.6,126
S$4213
  Bottom 0.152: 24.6,127 25.2,126.4
S$4214
  Bottom 0.152: 25.2,126.4 25.2,126
S$4215
  Bottom 0.152: 15.6,131 16.6,130
S$4216
  Bottom 0.152: 16.6,130 18,130
S$4217
  Bottom 0.152: 17.6,131 18,131
S$4218
  Bottom 0.152: 18,131 19,130
S$4219
  Bottom 0.152: 19,130 19.6,130
S$4220
  Bottom 0.152: 19.6,131 20.2,131
S$4221
  Bottom 0.152: 20.2,131 21.2,130
S$4222
  Bottom 0.152: 21.6,131 21.8,131
S$4223
  Bottom 0.152: 21.8,131 22.8,130
S$4224
  Bottom 0.152: 23.6,131 24.4,130.2
S$4225
  Bottom 0.152: 24.4,130.2 24.4,130
S$4226
  Bottom 0.152: 17.2,126 16,126
S$4227
  Bottom 0.152: 16,126 15,127
S$4228
  Bottom 0.152: 15,127 14.6,127
S$4229
  Bottom 0.152: 50.8,125 50.2,125
S$4230
  Bottom 0.152: 50.2,125 49.2,126
S$4231
  Bottom 0.152: 48.8,125 48.6,125
S$4232
  Bottom 0.152: 48.6,125 47.6,126
S$4233
  Bottom 0.152: 46.8,125 46,125.8
S$4234
  Bottom 0.152: 46,125.8 46,126
S$4235
  Bottom 0.152: 44.8,125 44.4,125.4
S$4236
  Bottom 0.152: 44.4,125.4 44.4,126
S$4237
  Bottom 0.152: 42.8,125 42.8,126
S$4238
  Bottom 0.152: 52.8,125 51.8,125
S$4239
  Bottom 0.152: 51.8,125 50.8,126
S$4240
  Bottom 0.152: 51.8,121 50.8,122
S$4241
  Bottom 0.152: 50.8,122 50,122
S$4242
  Bottom 0.152: 49.8,121 49.4,121
S$4243
  Bottom 0.152: 49.4,121 48.4,122
S$4244
  Bottom 0.152: 47.8,121 46.8,122
S$4245
  Bottom 0.152: 45.8,121 45.2,121.6
S$4246
  Bottom 0.152: 45.2,121.6 45.2,122
S$4247
  Bottom 0.152: 43.8,121 43.6,121.2
S$4248
  Bottom 0.152: 43.6,121.2 43.6,122
S$4249
  Bottom 0.152: 41.8,121 42,121.2
S$4250
  Bottom 0.152: 42,121.2 42,122
S$4251
  Bottom 0.152: 39.8,121 40.4,121.6
S$4252
  Bottom 0.152: 40.4,121.6 40.4,122
S$4253
  Bottom 0.152: 37.8,121 38.8,122
S$4254
  Bottom 0.152: 35.8,121 36.2,121
S$4255
  Bottom 0.152: 36.2,121 37.2,122
S$4256
  Bottom 0.152: 33.8,121 34.6,121
S$4257
  Bottom 0.152: 34.6,121 35.6,122
S$4258
  Bottom 0.152: 40.8,125 41.2,125.4
S$4259
  Bottom 0.152: 41.2,125.4 41.2,126
S$4260
  Bottom 0.152: 38.8,125 39.6,125.8
S$4261
  Bottom 0.152: 39.6,125.8 39.6,126
S$4262
  Bottom 0.152: 36.8,125 37,125
S$4263
  Bottom 0.152: 37,125 38,126
S$4264
  Bottom 0.152: 34.8,125 35.4,125
S$4265
  Bottom 0.152: 35.4,125 36.4,126
S$4266
  Bottom 0.152: 32.8,123 33.8,122
S$4267
  Bottom 0.152: 33.8,122 34.8,122
S$4268
  Bottom 0.152: 34.6,127 34,127
S$4269
  Bottom 0.152: 34,127 33,126
S$4270
  Bottom 0.152: 33,126 32.4,126
S$4271
  Bottom 0.152: 32.6,127 31.6,126
S$4272
  Bottom 0.152: 31.6,126 30.8,126
S$4273
  Bottom 0.152: 30.6,127 29.6,126
S$4274
  Bottom 0.152: 29.6,126 29.2,126
S$4275
  Bottom 0.152: 28.6,127 27.6,126
S$4276
  Bottom 0.152: 26.6,127 26,126.4
S$4277
  Bottom 0.152: 26,126.4 26,126
S$4278
  Bottom 0.152: 35.6,131 34.6,130
S$4279
  Bottom 0.152: 34.6,130 33.2,130
S$4280
  Bottom 0.152: 33.6,131 33.2,131
S$4281
  Bottom 0.152: 33.2,131 32.2,130
S$4282
  Bottom 0.152: 32.2,130 31.6,130
S$4283
  Bottom 0.152: 31.6,131 31,131
S$4284
  Bottom 0.152: 31,131 30,130
S$4285
  Bottom 0.152: 29.6,131 29.4,131
S$4286
  Bottom 0.152: 29.4,131 28.4,130
S$4287
  Bottom 0.152: 27.6,131 26.8,130.2
S$4288
  Bottom 0.152: 26.8,130.2 26.8,130
S$4289
  Bottom 0.152: 34,126 35.2,126
S$4290
  Bottom 0.152: 35.2,126 36.2,127
S$4291
  Bottom 0.152: 36.2,127 36.6,127
S$4292  (2 unrouted)
  Top 0.813: 65,130.5 65,121.5
  Top 1.8: 66,127.5 64,127.5 | 66,130.5 65,130.5 64,130.5 | 66,124.5 64,124.5 | 66,121.5 65,121.5 64,121.5
S$4293
  Top 1.778: -104.08,122.83 -104.08,124.35
S$4294
  Top 1.778: -104.08,127.65 -104.08,129.18
S$4295
  Top 1.778: -99,122.83 -99,124.35
S$4296
  Top 1.778: -99,127.65 -99,129.18
S$4297
  Top 1.778: -93.92,122.83 -93.92,124.35
S$4298
  Top 1.778: -93.92,127.65 -93.92,129.18
S$4299
  Top 1.778: 93.92,122.83 93.92,124.35
S$4300
  Top 1.778: 93.92,127.65 93.92,129.18
S$4301
  Top 1.778: 99,122.83 99,124.35
S$4302
  Top 1.778: 99,127.65 99,129.18
S$4303
  Top 1.778: 104.08,122.83 104.08,124.35
S$4304
  Top 1.778: 104.08,127.65 104.08,129.18
S$4313
  Bottom 0.8: 9.4,138.9 9.4,137.1
S$4314
  Bottom 0.8: 11.4,138.9 11.4,137.1
S$4315
  Bottom 0.8: 8.4,141.1 8.4,142.9
S$4316
  Bottom 0.8: 10.4,141.1 10.4,142.9
S$4317
  Bottom 0.8: 5.4,138.9 5.4,137.1
S$4318
  Bottom 0.8: 7.4,138.9 7.4,137.1
S$4319
  Bottom 0.8: 6.4,141.1 6.4,142.9
S$4320
  Bottom 0.8: 4.4,141.1 4.4,142.9
S$4321
  Bottom 0.8: 3.4,138.9 3.4,137.1
S$4322
  Bottom 0.8: 1.4,138.9 1.4,137.1
S$4323
  Bottom 0.8: 2.4,141.1 2.4,142.9
S$4324
  Bottom 0.8: 0.4,141.1 0.4,142.9
S$4325
  Bottom 0.8: -0.6,138.9 -0.6,137.1
S$4326
  Bottom 0.8: -2.6,138.9 -2.6,137.1
S$4327
  Bottom 0.8: -1.6,141.1 -1.6,142.9
S$4328
  Bottom 0.8: 17.4,138.9 17.4,137.1
S$4329
  Bottom 0.8: 19.4,138.9 19.4,137.1
S$4330
  Bottom 0.8: 16.4,141.1 16.4,142.9
S$4331
  Bottom 0.8: 18.4,141.1 18.4,142.9
S$4332
  Bottom 0.8: 13.4,138.9 13.4,137.1
S$4333
  Bottom 0.8: 15.4,138.9 15.4,137.1
S$4334
  Bottom 0.8: 12.4,141.1 12.4,142.9
S$4335
  Bottom 0.8: 14.4,141.1 14.4,142.9
S$4336
  Bottom 0.8: -7.4,146.9 -7.4,145.1
S$4337
  Bottom 0.8: -5.4,146.9 -5.4,145.1
S$4338
  Bottom 0.8: -8.4,149.1 -8.4,150.9
S$4339
  Bottom 0.8: -6.4,149.1 -6.4,150.9
S$4340
  Bottom 0.8: -11.4,146.9 -11.4,145.1
S$4341
  Bottom 0.8: -9.4,146.9 -9.4,145.1
S$4342
  Bottom 0.8: -10.4,149.1 -10.4,150.9
S$4343
  Bottom 0.8: -12.4,149.1 -12.4,150.9
S$4344
  Bottom 0.8: -13.4,146.9 -13.4,145.1
S$4345
  Bottom 0.8: -15.4,146.9 -15.4,145.1
S$4346
  Bottom 0.8: -14.4,149.1 -14.4,150.9
S$4347
  Bottom 0.8: -16.4,149.1 -16.4,150.9
S$4348
  Bottom 0.8: -17.4,146.9 -17.4,145.1
S$4349
  Bottom 0.8: -19.4,146.9 -19.4,145.1
S$4350
  Bottom 0.8: -18.4,149.1 -18.4,150.9
S$4351
  Bottom 0.8: 0.6,146.9 0.6,145.1
S$4352
  Bottom 0.8: 2.6,146.9 2.6,145.1
S$4353
  Bottom 0.8: -0.4,149.1 -0.4,150.9
S$4354
  Bottom 0.8: 1.6,149.1 1.6,150.9
S$4355
  Bottom 0.8: -3.4,146.9 -3.4,145.1
S$4356
  Bottom 0.8: -1.4,146.9 -1.4,145.1
S$4357
  Bottom 0.8: -4.4,149.1 -4.4,150.9
S$4358
  Bottom 0.8: -2.4,149.1 -2.4,150.9
S$4359
  Bottom 0.8: -24.6,138.9 -24.6,137.1
S$4360
  Bottom 0.8: -22.6,138.9 -22.6,137.1
S$4361
  Bottom 0.8: -25.6,141.1 -25.6,142.9
S$4362
  Bottom 0.8: -23.6,141.1 -23.6,142.9
S$4363
  Bottom 0.8: -28.6,138.9 -28.6,137.1
S$4364
  Bottom 0.8: -26.6,138.9 -26.6,137.1
S$4365
  Bottom 0.8: -27.6,141.1 -27.6,142.9
S$4366
  Bottom 0.8: -29.6,141.1 -29.6,142.9
S$4367
  Bottom 0.8: -30.6,138.9 -30.6,137.1
S$4368
  Bottom 0.8: -32.6,138.9 -32.6,137.1
S$4369
  Bottom 0.8: -31.6,141.1 -31.6,142.9
S$4370
  Bottom 0.8: -33.6,141.1 -33.6,142.9
S$4371
  Bottom 0.8: -34.6,138.9 -34.6,137.1
S$4372
  Bottom 0.8: -36.6,138.9 -36.6,137.1
S$4373
  Bottom 0.8: -35.6,141.1 -35.6,142.9
S$4374
  Bottom 0.8: -16.6,138.9 -16.6,137.1
S$4375
  Bottom 0.8: -14.6,138.9 -14.6,137.1
S$4376
  Bottom 0.8: -17.6,141.1 -17.6,142.9
S$4377
  Bottom 0.8: -15.6,141.1 -15.6,142.9
S$4378
  Bottom 0.8: -20.6,138.9 -20.6,137.1
S$4379
  Bottom 0.8: -18.6,138.9 -18.6,137.1
S$4380
  Bottom 0.8: -21.6,141.1 -21.6,142.9
S$4381
  Bottom 0.8: -19.6,141.1 -19.6,142.9
S$4382
  Bottom 0.8: 26.6,146.9 26.6,145.1
S$4383
  Bottom 0.8: 28.6,146.9 28.6,145.1
S$4384
  Bottom 0.8: 25.6,149.1 25.6,150.9
S$4385
  Bottom 0.8: 27.6,149.1 27.6,150.9
S$4386
  Bottom 0.8: 22.6,146.9 22.6,145.1
S$4387
  Bottom 0.8: 24.6,146.9 24.6,145.1
S$4388
  Bottom 0.8: 23.6,149.1 23.6,150.9
S$4389
  Bottom 0.8: 21.6,149.1 21.6,150.9
S$4390
  Bottom 0.8: 20.6,146.9 20.6,145.1
S$4391
  Bottom 0.8: 18.6,146.9 18.6,145.1
S$4392
  Bottom 0.8: 19.6,149.1 19.6,150.9
S$4393
  Bottom 0.8: 17.6,149.1 17.6,150.9
S$4394
  Bottom 0.8: 16.6,146.9 16.6,145.1
S$4395
  Bottom 0.8: 14.6,146.9 14.6,145.1
S$4396
  Bottom 0.8: 15.6,149.1 15.6,150.9
S$4397
  Bottom 0.8: 34.6,146.9 34.6,145.1
S$4398
  Bottom 0.8: 36.6,146.9 36.6,145.1
S$4399
  Bottom 0.8: 33.6,149.1 33.6,150.9
S$4400
  Bottom 0.8: 35.6,149.1 35.6,150.9
S$4401
  Bottom 0.8: 30.6,146.9 30.6,145.1
S$4402
  Bottom 0.8: 32.6,146.9 32.6,145.1
S$4403
  Bottom 0.8: 29.6,149.1 29.6,150.9
S$4404
  Bottom 0.8: 31.6,149.1 31.6,150.9
S$4405
  Bottom 0.8: -41.8,146.9 -41.8,145.1
S$4406
  Bottom 0.8: -39.8,146.9 -39.8,145.1
S$4407
  Bottom 0.8: -42.8,149.1 -42.8,150.9
S$4408
  Bottom 0.8: -40.8,149.1 -40.8,150.9
S$4409
  Bottom 0.8: -45.8,146.9 -45.8,145.1
S$4410
  Bottom 0.8: -43.8,146.9 -43.8,145.1
S$4411
  Bottom 0.8: -44.8,149.1 -44.8,150.9
S$4412
  Bottom 0.8: -46.8,149.1 -46.8,150.9
S$4413
  Bottom 0.8: -47.8,146.9 -47.8,145.1
S$4414
  Bottom 0.8: -49.8,146.9 -49.8,145.1
S$4415
  Bottom 0.8: -48.8,149.1 -48.8,150.9
S$4416
  Bottom 0.8: -50.8,149.1 -50.8,150.9
S$4417
  Bottom 0.8: -51.8,146.9 -51.8,145.1
S$4418
  Bottom 0.8: -53.8,146.9 -53.8,145.1
S$4419
  Bottom 0.8: -52.8,149.1 -52.8,150.9
S$4420
  Bottom 0.8: -33.8,146.9 -33.8,145.1
S$4421
  Bottom 0.8: -31.8,146.9 -31.8,145.1
S$4422
  Bottom 0.8: -34.8,149.1 -34.8,150.9
S$4423
  Bottom 0.8: -32.8,149.1 -32.8,150.9
S$4424
  Bottom 0.8: -37.8,146.9 -37.8,145.1
S$4425
  Bottom 0.8: -35.8,146.9 -35.8,145.1
S$4426
  Bottom 0.8: -38.8,149.1 -38.8,150.9
S$4427
  Bottom 0.8: -36.8,149.1 -36.8,150.9
S$4428
  Bottom 0.8: 43.8,138.9 43.8,137.1
S$4429
  Bottom 0.8: 45.8,138.9 45.8,137.1
S$4430
  Bottom 0.8: 42.8,141.1 42.8,142.9
S$4431
  Bottom 0.8: 44.8,141.1 44.8,142.9
S$4432
  Bottom 0.8: 39.8,138.9 39.8,137.1
S$4433
  Bottom 0.8: 41.8,138.9 41.8,137.1
S$4434
  Bottom 0.8: 40.8,141.1 40.8,142.9
S$4435
  Bottom 0.8: 38.8,141.1 38.8,142.9
S$4436
  Bottom 0.8: 37.8,138.9 37.8,137.1
S$4437
  Bottom 0.8: 35.8,138.9 35.8,137.1
S$4438
  Bottom 0.8: 36.8,141.1 36.8,142.9
S$4439
  Bottom 0.8: 34.8,141.1 34.8,142.9
S$4440
  Bottom 0.8: 33.8,138.9 33.8,137.1
S$4441
  Bottom 0.8: 31.8,138.9 31.8,137.1
S$4442
  Bottom 0.8: 32.8,141.1 32.8,142.9
S$4443
  Bottom 0.8: 51.8,138.9 51.8,137.1
S$4444
  Bottom 0.8: 53.8,138.9 53.8,137.1
S$4445
  Bottom 0.8: 50.8,141.1 50.8,142.9
S$4446
  Bottom 0.8: 52.8,141.1 52.8,142.9
S$4447
  Bottom 0.8: 47.8,138.9 47.8,137.1
S$4448
  Bottom 0.8: 49.8,138.9 49.8,137.1
S$4449
  Bottom 0.8: 46.8,141.1 46.8,142.9
S$4450
  Bottom 0.8: 48.8,141.1 48.8,142.9
S$4579
  Bottom 0.152: -52.8,149 -51.8,148
S$4580
  Bottom 0.152: -51.8,148 -50.8,148
S$4581
  Bottom 0.152: -50.8,149 -50.2,149
S$4582
  Bottom 0.152: -50.2,149 -49.2,148
S$4583
  Bottom 0.152: -48.8,149 -48.6,149
S$4584
  Bottom 0.152: -48.6,149 -47.6,148
S$4585
  Bottom 0.152: -46.8,149 -46,148.2
S$4586
  Bottom 0.152: -46,148.2 -46,148
S$4587
  Bottom 0.152: -44.8,149 -44.4,148.6
S$4588
  Bottom 0.152: -44.4,148.6 -44.4,148
S$4589
  Bottom 0.152: -42.8,149 -42.8,148
S$4590
  Bottom 0.152: -40.8,149 -41.2,148.6
S$4591
  Bottom 0.152: -41.2,148.6 -41.2,148
S$4592
  Bottom 0.152: -38.8,149 -39.6,148.2
S$4593
  Bottom 0.152: -39.6,148.2 -39.6,148
S$4594
  Bottom 0.152: -36.8,149 -37,149
S$4595
  Bottom 0.152: -37,149 -38,148
S$4596
  Bottom 0.152: -34.8,149 -35.4,149
S$4597
  Bottom 0.152: -35.4,149 -36.4,148
S$4598
  Bottom 0.152: -32.8,149 -33.8,148
S$4599
  Bottom 0.152: -33.8,148 -34.8,148
S$4600
  Bottom 0.152: -51.8,145 -50.8,144
S$4601
  Bottom 0.152: -50.8,144 -50,144
S$4602
  Bottom 0.152: -49.8,145 -48.8,144
S$4603
  Bottom 0.152: -48.8,144 -48.4,144
S$4604
  Bottom 0.152: -47.8,145 -46.8,144
S$4605
  Bottom 0.152: -45.8,145 -45.2,144.4
S$4606
  Bottom 0.152: -45.2,144.4 -45.2,144
S$4607
  Bottom 0.152: -43.8,145 -43.6,144.8
S$4608
  Bottom 0.152: -43.6,144.8 -43.6,144
S$4609
  Bottom 0.152: -41.8,145 -42,144.8
S$4610
  Bottom 0.152: -42,144.8 -42,144
S$4611
  Bottom 0.152: -39.8,145 -40.4,144.4
S$4612
  Bottom 0.152: -40.4,144.4 -40.4,144
S$4613
  Bottom 0.152: -37.8,145 -38.8,144
S$4614
  Bottom 0.152: -35.8,145 -36.8,144
S$4615
  Bottom 0.152: -36.8,144 -37.2,144
S$4616
  Bottom 0.152: -33.8,145 -34.8,144
S$4617
  Bottom 0.152: -34.8,144 -35.6,144
S$4618
  Bottom 0.152: -36.6,139 -35.6,140
S$4619
  Bottom 0.152: -35.6,140 -34,140
S$4620
  Bottom 0.152: -34.6,139 -33.8,139
S$4621
  Bottom 0.152: -33.8,139 -32.8,140
S$4622
  Bottom 0.152: -32.8,140 -32.4,140
S$4623
  Bottom 0.152: -32.6,139 -31.8,139
S$4624
  Bottom 0.152: -31.8,139 -30.8,140
S$4625
  Bottom 0.152: -30.6,139 -30.2,139
S$4626
  Bottom 0.152: -30.2,139 -29.2,140
S$4627
  Bottom 0.152: -28.6,139 -27.6,140
S$4628
  Bottom 0.152: -26.6,139 -26,139.6
S$4629
  Bottom 0.152: -26,139.6 -26,140
S$4630
  Bottom 0.152: -35.6,143 -35,143
S$4631
  Bottom 0.152: -35,143 -34,144
S$4632
  Bottom 0.152: -34,144 -33.2,144
S$4633
  Bottom 0.152: -33.6,143 -33,143
S$4634
  Bottom 0.152: -33,143 -32,144
S$4635
  Bottom 0.152: -32,144 -31.6,144
S$4636
  Bottom 0.152: -31.6,143 -31,143
S$4637
  Bottom 0.152: -31,143 -30,144
S$4638
  Bottom 0.152: -29.6,143 -29.4,143
S$4639
  Bottom 0.152: -29.4,143 -28.4,144
S$4640
  Bottom 0.152: -27.6,143 -26.8,143.8
S$4641
  Bottom 0.152: -26.8,143.8 -26.8,144
S$4642
  Bottom 0.152: 1.6,149 0.6,148
S$4643
  Bottom 0.152: 0.6,148 -0.4,148
S$4644
  Bottom 0.152: -0.4,149 -1,149
S$4645
  Bottom 0.152: -1,149 -2,148
S$4646
  Bottom 0.152: -2.4,149 -2.6,149
S$4647
  Bottom 0.152: -2.6,149 -3.6,148
S$4648
  Bottom 0.152: -4.4,149 -5.2,148.2
S$4649
  Bottom 0.152: -5.2,148.2 -5.2,148
S$4650
  Bottom 0.152: -6.4,149 -6.8,148.6
S$4651
  Bottom 0.152: -6.8,148.6 -6.8,148
S$4652
  Bottom 0.152: -8.4,149 -8.4,148
S$4653
  Bottom 0.152: -10.4,149 -10,148.6
S$4654
  Bottom 0.152: -10,148.6 -10,148
S$4655
  Bottom 0.152: -12.4,149 -11.6,148.2
S$4656
  Bottom 0.152: -11.6,148.2 -11.6,148
S$4657
  Bottom 0.152: -14.4,149 -14.2,149
S$4658
  Bottom 0.152: -14.2,149 -13.2,148
S$4659
  Bottom 0.152: -16.4,149 -15.8,149
S$4660
  Bottom 0.152: -15.8,149 -14.8,148
S$4661
  Bottom 0.152: -18.4,149 -17.4,148
S$4662
  Bottom 0.152: -17.4,148 -16.4,148
S$4663
  Bottom 0.152: 0.6,145 -0.4,144
S$4664
  Bottom 0.152: -0.4,144 -1.2,144
S$4665
  Bottom 0.152: -1.4,145 -2.4,144
S$4666
  Bottom 0.152: -2.4,144 -2.8,144
S$4667
  Bottom 0.152: -3.4,145 -4.4,144
S$4668
  Bottom 0.152: -5.4,145 -6,144.4
S$4669
  Bottom 0.152: -6,144.4 -6,144
S$4670
  Bottom 0.152: -7.4,145 -7.6,144.8
S$4671
  Bottom 0.152: -7.6,144.8 -7.6,144
S$4672
  Bottom 0.152: -9.4,145 -9.2,144.8
S$4673
  Bottom 0.152: -9.2,144.8 -9.2,144
S$4674
  Bottom 0.152: -11.4,145 -10.8,144.4
S$4675
  Bottom 0.152: -10.8,144.4 -10.8,144
S$4676
  Bottom 0.152: -13.4,145 -12.4,144
S$4677
  Bottom 0.152: -15.4,145 -14.4,144
S$4678
  Bottom 0.152: -14.4,144 -14,144
S$4679
  Bottom 0.152: -17.4,145 -16.4,144
S$4680
  Bottom 0.152: -16.4,144 -15.6,144
S$4681
  Bottom 0.152: -14.6,139 -15.6,140
S$4682
  Bottom 0.152: -15.6,140 -17.2,140
S$4683
  Bottom 0.152: -16.6,139 -17.4,139
S$4684
  Bottom 0.152: -17.4,139 -18.4,140
S$4685
  Bottom 0.152: -18.4,140 -18.8,140
S$4686
  Bottom 0.152: -18.6,139 -19.4,139
S$4687
  Bottom 0.152: -19.4,139 -20.4,140
S$4688
  Bottom 0.152: -20.6,139 -21,139
S$4689
  Bottom 0.152: -21,139 -22,140
S$4690
  Bottom 0.152: -22.6,139 -23.6,140
S$4691
  Bottom 0.152: -24.6,139 -25.2,139.6
S$4692
  Bottom 0.152: -25.2,139.6 -25.2,140
S$4693
  Bottom 0.152: -15.6,143 -16.2,143
S$4694
  Bottom 0.152: -16.2,143 -17.2,144
S$4695
  Bottom 0.152: -17.2,144 -18,144
S$4696
  Bottom 0.152: -17.6,143 -18.2,143
S$4697
  Bottom 0.152: -18.2,143 -19.2,144
S$4698
  Bottom 0.152: -19.2,144 -19.6,144
S$4699
  Bottom 0.152: -19.6,143 -20.2,143
S$4700
  Bottom 0.152: -20.2,143 -21.2,144
S$4701
  Bottom 0.152: -21.6,143 -21.8,143
S$4702
  Bottom 0.152: -21.8,143 -22.8,144
S$4703
  Bottom 0.152: -23.6,143 -24.4,143.8
S$4704
  Bottom 0.152: -24.4,143.8 -24.4,144
S$4705
  Bottom 0.152: 0.4,143 1,143
S$4706
  Bottom 0.152: 1,143 2,144
S$4707
  Bottom 0.152: 2.4,143 2.6,143
S$4708
  Bottom 0.152: 2.6,143 3.6,144
S$4709
  Bottom 0.152: 4.4,143 5.2,143.8
S$4710
  Bottom 0.152: 5.2,143.8 5.2,144
S$4711
  Bottom 0.152: 6.4,143 6.8,143.4
S$4712
  Bottom 0.152: 6.8,143.4 6.8,144
S$4713
  Bottom 0.152: 8.4,143 8.4,144
S$4714
  Bottom 0.152: -1.6,143 -0.6,143
S$4715
  Bottom 0.152: -0.6,143 0.4,144
S$4716
  Bottom 0.152: -0.6,139 0.4,140
S$4717
  Bottom 0.152: 0.4,140 1.2,140
S$4718
  Bottom 0.152: 1.4,139 1.8,139
S$4719
  Bottom 0.152: 1.8,139 2.8,140
S$4720
  Bottom 0.152: 3.4,139 4.4,140
S$4721
  Bottom 0.152: 5.4,139 6,139.6
S$4722
  Bottom 0.152: 6,139.6 6,140
S$4723
  Bottom 0.152: 7.4,139 7.6,139.2
S$4724
  Bottom 0.152: 7.6,139.2 7.6,140
S$4725
  Bottom 0.152: 9.4,139 9.2,139.2
S$4726
  Bottom 0.152: 9.2,139.2 9.2,140
S$4727
  Bottom 0.152: 11.4,139 10.8,139.6
S$4728
  Bottom 0.152: 10.8,139.6 10.8,140
S$4729
  Bottom 0.152: 13.4,139 12.4,140
S$4730
  Bottom 0.152: 15.4,139 15,139
S$4731
  Bottom 0.152: 15,139 14,140
S$4732
  Bottom 0.152: 17.4,139 16.6,139
S$4733
  Bottom 0.152: 16.6,139 15.6,140
S$4734
  Bottom 0.152: 10.4,143 10,143.4
S$4735
  Bottom 0.152: 10,143.4 10,144
S$4736
  Bottom 0.152: 12.4,143 11.6,143.8
S$4737
  Bottom 0.152: 11.6,143.8 11.6,144
S$4738
  Bottom 0.152: 14.4,143 14.2,143
S$4739
  Bottom 0.152: 14.2,143 13.2,144
S$4740
  Bottom 0.152: 16.4,143 15.8,143
S$4741
  Bottom 0.152: 15.8,143 14.8,144
S$4742
  Bottom 0.152: 18.4,141 17.4,140
S$4743
  Bottom 0.152: 17.4,140 16.4,140
S$4744
  Bottom 0.152: 16.6,145 17.2,145
S$4745
  Bottom 0.152: 17.2,145 18.2,144
S$4746
  Bottom 0.152: 18.2,144 18.8,144
S$4747
  Bottom 0.152: 18.6,145 19.6,144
